PROGRAM MAIN
VAR
	array10 AT %I*: ARRAY [0..9] OF INT;  //声明采集回的数组变量
	array20:ARRAY[0..9] OF LREAL;         //声明处理过后的数组变量
END_VAR

array20[0]:=INT_TO_LREAL (array10[0]);
array20[1]:=INT_TO_LREAL (array10[1]);
array20[2]:=INT_TO_LREAL (array10[2]);
array20[3]:=INT_TO_LREAL (array10[3]);
array20[4]:=INT_TO_LREAL (array10[4]);
array20[5]:=INT_TO_LREAL (array10[5]);
array20[6]:=INT_TO_LREAL (array10[6]);
array20[7]:=INT_TO_LREAL (array10[7]);
array20[8]:=INT_TO_LREAL (array10[8]);
array20[9]:=INT_TO_LREAL (array10[9]);      //将数组中的元素从INT类型转换至LREAL类型

array20[0]:=array20[0]/3276.7;
array20[1]:=array20[1]/3276.7;
array20[2]:=array20[2]/3276.7;
array20[3]:=array20[3]/3276.7;
array20[4]:=array20[4]/3276.7;
array20[5]:=array20[5]/3276.7;
array20[6]:=array20[6]/3276.7;
array20[7]:=array20[7]/3276.7;
array20[8]:=array20[8]/3276.7;
array20[9]:=array20[9]/3276.7;              //处理传输回的数据

END_PROGRAM
